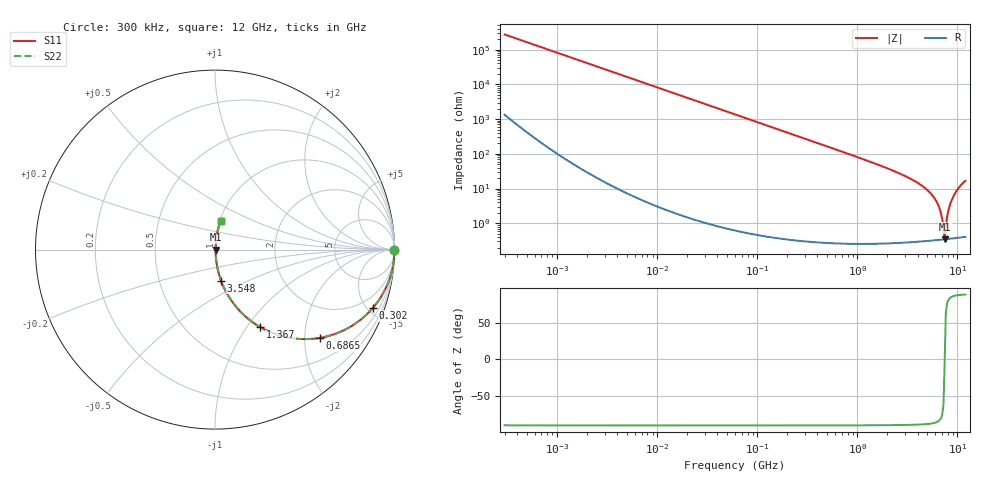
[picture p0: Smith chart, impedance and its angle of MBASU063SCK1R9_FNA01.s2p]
! MBASU063SCK1R9_FNA01  S-PARAMETER MODEL  ( General Type )
! Model Generated by TAIYO YUDEN Corporation (http://www.ty-top.com)
! Version 1.0
! TAIYO YUDEN Control No. 130801
! Copyright(c) 2013 TAIYO YUDEN CO.,LTD. All Rights Reserved.
! Product Description (link to TY-COMPAS)
! https://ds.yuden.co.jp/TYCOMPAS/or/detail?pn=MBASU063SCK1R9CFNA01&u=M
! Products Name : Multilayer Ceramic Capacitors
! Characteristics :
!  Capacitance : 1.9 pF , Rated Voltage : 50V , TCC : CK / C0K
!  Case Size : 0.6 x 0.3 / 0.024 x 0.012 [mm/inch] , Thickness : 0.3 / 0.012 [mm/inch]
!  (Conditions: Temperature = 25 degC , DC Bias Current/Voltage = 0A / 0V)
! External Node Assignments :
!  1  o---| |---o  2
! GND o---------o GND
! Frequency Range : 0.3MHz  -  12000MHz  [ 401 STEP ]
# MHz S RI R 50
! Freq[MHz].  S11 Real  S11 Imag  S21 Real  S21 Imag  S12 Real  S12 Imag  S22 Real  S22 Imag
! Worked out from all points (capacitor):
!   401 points, 300 kHz to 12 GHz, reference 50 ohm
!   read as one part in series: C = 1.94 pF near 316.3 kHz
!   lowest |Z| = 347 mohm at 7.449 GHz (marker M1)
!   series resonance near 7.455 GHz, so ESL is about 240 pH
!   S11 on the Smith chart (normalised r, x): 300 kHz: open; 302 MHz: 1.01, -5.43; 686.5 MHz: 1.01, -2.37; 1.367 GHz: 1.01, -1.16; 3.548 GHz: 1.01, -0.36; 12 GHz: 1.01, +0.33
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0.3  1 -0.000365  1.92e-06 0.000365  1.92e-06 0.000365  1 -0.000365
1.769972  1 -0.00216  6.32e-06 0.00216  6.32e-06 0.00216  1 -0.00216
10.44266  0.9998 -0.0127  0.000167 0.0127  0.000167 0.0127  0.9998 -0.0127
60  0.9947 -0.0727  0.00535 0.0727  0.00535 0.0727  0.9947 -0.0727
301.9711  0.8802 -0.3242  0.1198 0.3242  0.1198 0.3242  0.8802 -0.3242
353.9943  0.8423 -0.3639  0.1577 0.3639  0.1577 0.3639  0.8423 -0.3639
686.4755  0.5841 -0.4918  0.4159 0.4918  0.4159 0.4918  0.5841 -0.4918
1366.97  0.2529 -0.4325  0.7471 0.4325  0.7471 0.4325  0.2529 -0.4325
2088.533  0.1178 -0.3187  0.8822 0.3187  0.8822 0.3187  0.1178 -0.3187
3547.679  0.0337 -0.1726  0.9663 0.1726  0.9663 0.1726  0.0337 -0.1726
4747.894  0.0134 -0.1012  0.9866 0.1012  0.9866 0.1012  0.0134 -0.1012
5868.704  0.00603 -0.0529  0.994 0.0529  0.994 0.0529  0.00603 -0.0529
6524.734  0.00419 -0.0294  0.9958 0.0294  0.9958 0.0294  0.00419 -0.0294
6879.757  0.00369 -0.0178  0.9963 0.0178  0.9963 0.0178  0.00369 -0.0178
7064.448  0.00354 -0.012  0.9965 0.012  0.9965 0.012  0.00354 -0.012
7254.098  0.00346 -0.00621  0.9965 0.00621  0.9965 0.00621  0.00346 -0.00621
7448.838  0.00345 -0.000221  0.9966 0.000221  0.9966 0.000221  0.00345 -0.000221
7648.807  0.00352 0.00675  0.9965 -0.00675  0.9965 -0.00675  0.00352 0.00675
8281.503  0.00439 0.0286  0.9956 -0.0286  0.9956 -0.0286  0.00439 0.0286
8966.534  0.00654 0.0535  0.9935 -0.0535  0.9935 -0.0535  0.00654 0.0535
10236.47  0.0142 0.1011  0.9858 -0.1011  0.9858 -0.1011  0.0142 0.1011
12000  0.0308 0.1609  0.9692 -0.1609  0.9692 -0.1609  0.0308 0.1609
